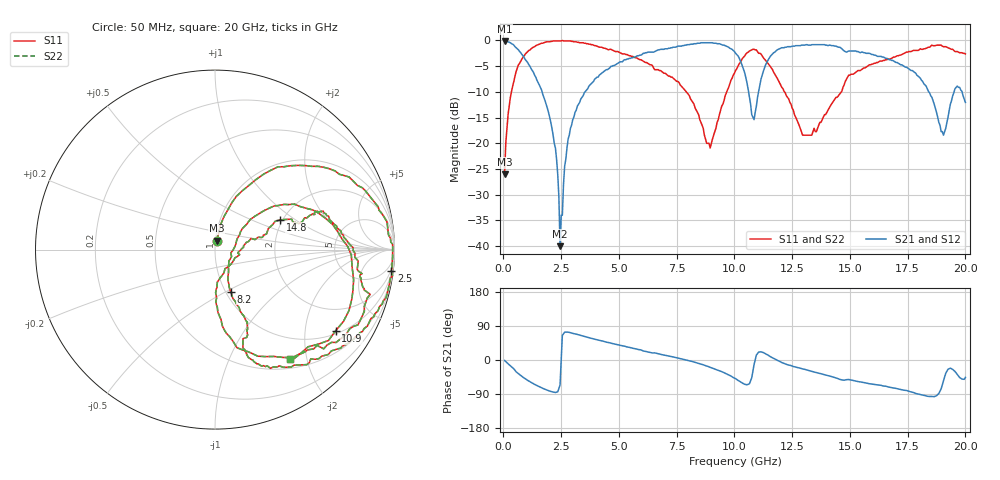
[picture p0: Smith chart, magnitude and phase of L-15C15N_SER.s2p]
# MHZ S MA R 50
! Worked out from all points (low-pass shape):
!   400 points, 50 MHz to 20 GHz, reference 50 ohm
!   highest |S21| = -0.09 dB at 50 MHz (marker M1); lowest = -40.0 dB at 2.45 GHz (marker M2)
!   |S21| within 3 dB of the highest: 5.754 GHz to 10.16 GHz (4.411 GHz wide, 55.4 % of centre); 11.55 GHz to 16.2 GHz (4.643 GHz wide, 33.5 % of centre)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
!   lowest |S11| = -26.0 dB at 50 MHz (marker M3), VSWR 1.11, Z = 50.8 + j4.98 ohm
!   |S11| at or under -10 dB: start of sweep to 345.6 MHz; 7.919 GHz to 9.666 GHz (1.747 GHz wide, 19.9 % of centre); 12.17 GHz to 14.63 GHz (2.463 GHz wide, 18.4 % of centre)
!   |S22| runs from -26.0 to 0.0 dB; largest |S21 - S12| = 0
!   S11 on the Smith chart (normalised r, x): 50 MHz: 1.02, +0.10; 2.5 GHz: 1, -16; 8.2 GHz: 1.06, -0.53; 10.9 GHz: 1.10, -2.89; 14.8 GHz: 1.95, +0.77; 20 GHz: 0.63, -1.71
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50  0.05 77.8  0.99 -1.2  0.99 -1.2  0.05 77.8
200  0.19 74.8  0.97 -9.9  0.97 -9.9  0.19 74.8
550  0.5 57.2  0.85 -31.2  0.85 -31.2  0.5 57.2
1950  0.97 6.2  0.2 -80.9  0.2 -80.9  0.97 6.2
2300  0.99 -2.3  0.07 -84.9  0.07 -84.9  0.99 -2.3
2450  0.99 -5.5  0.01 -66.1  0.01 -66.1  0.99 -5.5
2500  0.99 -6.9  0.02 -0.6  0.02 -0.6  0.99 -6.9
2800  0.99 -13.5  0.11 73.2  0.11 73.2  0.99 -13.5
3400  0.95 -25.6  0.28 64.0  0.28 64.0  0.95 -25.6
6700  0.52 -70.1  0.81 16.4  0.81 16.4  0.52 -70.1
8200  0.25 -69.6  0.92 -4.4  0.92 -4.4  0.25 -69.6
8950  0.09 -11.4  0.95 -19.4  0.95 -19.4  0.09 -11.4
10050  0.51 29.8  0.75 -49.1  0.75 -49.1  0.51 29.8
10900  0.81 -34.0  0.2 0.5  0.2 0.5  0.81 -34.0
11750  0.47 -82.3  0.77 2.4  0.77 2.4  0.47 -82.3
13350  0.12 -22.8  0.91 -29.9  0.91 -29.9  0.12 -22.8
14800  0.4 24.4  0.78 -52.6  0.78 -52.6  0.4 24.4
16700  0.66 15.5  0.65 -71.6  0.65 -71.6  0.66 15.5
18300  0.84 -13.0  0.36 -94.7  0.36 -94.7  0.84 -13.0
19050  0.87 -30.6  0.12 -55.0  0.12 -55.0  0.87 -30.6
19550  0.78 -43.2  0.34 -30.3  0.34 -30.3  0.78 -43.2
20000  0.74 -55.8  0.25 -45.9  0.25 -45.9  0.74 -55.8
